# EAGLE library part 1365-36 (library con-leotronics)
DUAL ROW STRAIGHT HEADER 1364 SERIES. 1.27mm x 1.27mm. Without Fixing Post. SMT Source: http://www.leotronics.co.uk/Conexcon/Data%20Sheets/sec.%20A/1364ing.pdf
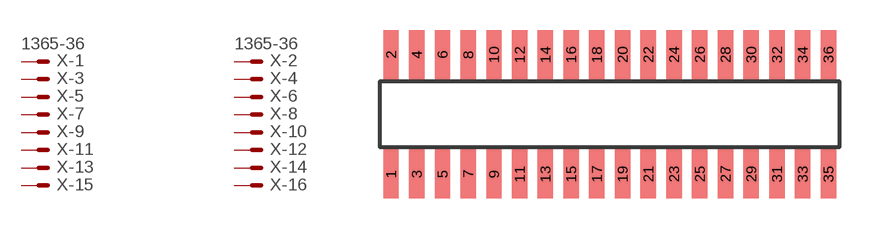
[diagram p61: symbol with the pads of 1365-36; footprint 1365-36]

Designator prefix X; gates -1=MVAL -2=MVAL -3=M -4=M -5=M -6=M -7=M -8=M -9=M -10=M -11=M -12=M -13=M -14=M -15=M -16=M -17=M -18=M -19=M -20=M -21=M -22=M -23=M -24=M -25=M -26=M -27=M -28=M -29=M -30=M -31=M -32=M -33=M -34=M -35=M -36=M

## 1365-36 (OC_FARNELL: unknown; OC_NEWARK: unknown)  [1365-36]
1  -1:S  pas
2  -2:S  pas
3  -3:S  pas
4  -4:S  pas
5  -5:S  pas
6  -6:S  pas
7  -7:S  pas
8  -8:S  pas
9  -9:S  pas
10  -10:S  pas
11  -11:S  pas
12  -12:S  pas
13  -13:S  pas
14  -14:S  pas
15  -15:S  pas
16  -16:S  pas
17  -17:S  pas
18  -18:S  pas
19  -19:S  pas
20  -20:S  pas
21  -21:S  pas
22  -22:S  pas
23  -23:S  pas
24  -24:S  pas
25  -25:S  pas
26  -26:S  pas
27  -27:S  pas
28  -28:S  pas
29  -29:S  pas
30  -30:S  pas
31  -31:S  pas
32  -32:S  pas
33  -33:S  pas
34  -34:S  pas
35  -35:S  pas
36  -36:S  pas

## Footprint 1365-36 (pad centres in mm)
DUAL ROW STRAIGHT HEADER 1364 SERIES. 1.27mm x 1.27mm. Without Fixing Post. SMT Source: http://www.leotronics.co.uk/Conexcon/Data%20Sheets/sec.%20A/1364ing.pdf
smd 0.76 x 2.4: 1 -10.795,-2.95; 2 -10.795,2.95; 3 -9.525,-2.95; 4 -9.525,2.95; 5 -8.255,-2.95; 6 -8.255,2.95; 7 -6.985,-2.95; 8 -6.985,2.95; 9 -5.715,-2.95; 10 -5.715,2.95; 11 -4.445,-2.95; 12 -4.445,2.95; 13 -3.175,-2.95; 14 -3.175,2.95; 15 -1.905,-2.95; 16 -1.905,2.95; 17 -0.635,-2.95; 18 -0.635,2.95; 19 0.635,-2.95; 20 0.635,2.95; 21 1.905,-2.95; 22 1.905,2.95; 23 3.175,-2.95; 24 3.175,2.95; 25 4.445,-2.95; 26 4.445,2.95; 27 5.715,-2.95; 28 5.715,2.95; 29 6.985,-2.95; 30 6.985,2.95; 31 8.255,-2.95; 32 8.255,2.95; 33 9.525,-2.95; 34 9.525,2.95; 35 10.795,-2.95; 36 10.795,2.95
